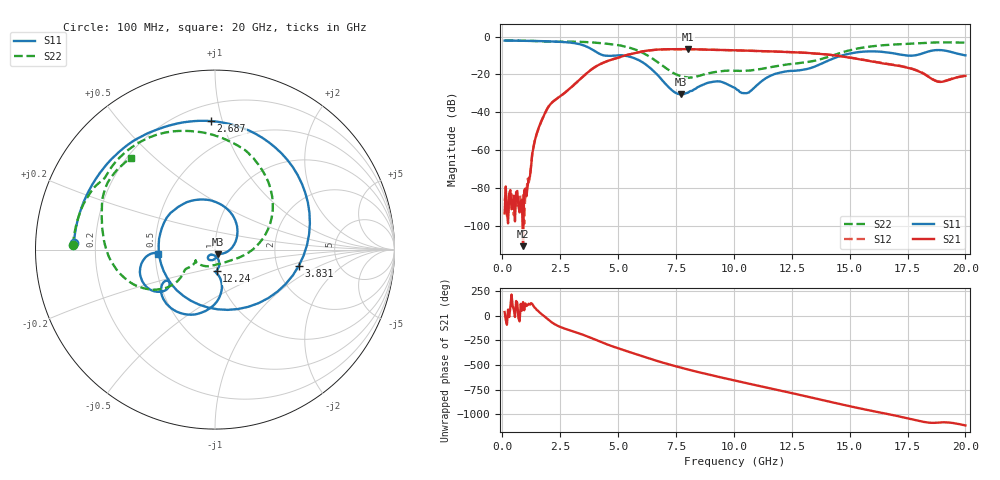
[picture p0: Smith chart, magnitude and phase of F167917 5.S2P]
!  2-Port S-parameters saved by WinCal
! VAR MeasName=S-Parameters (CALIBRATED_DATA) read from VNA (N5242A)
! VAR MeasDate=2016-11-22 8:59:55
! VAR NAME=F167917 5
! VAR FILENAME=F167917 5.S2P
! VAR DATE=2016-11-22 8:59:55
! VAR PHYS_PORTS=1,2
# Hz S DB R 50
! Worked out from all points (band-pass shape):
!   401 points, 100 MHz to 20 GHz, reference 50 ohm
!   highest |S21| = -6.61 dB at 8.01 GHz (marker M1); lowest = -110.9 dB at 896 MHz (marker M2)
!   |S21| within 3 dB of the highest: 5.422 GHz to 14.12 GHz (8.699 GHz wide, 89 % of centre)
!   lowest |S11| = -30.6 dB at 7.712 GHz (marker M3), VSWR 1.06, Z = 51.5 - j2.6 ohm
!   |S11| at or under -10 dB: 4.415 GHz to 4.905 GHz (490 MHz wide, 10.5 % of centre); 5.227 GHz to 14.66 GHz (9.438 GHz wide, 94.9 % of centre); 17.47 GHz to 17.77 GHz (294.6 MHz wide, 1.67 % of centre)
!   |S22| runs from -21.8 to -2.0 dB; largest |S21 - S12| = 0.0047
!   S11 on the Smith chart (normalised r, x): 100 MHz: 0.12, +0.02; 2.687 GHz: 0.31, +0.92; 3.831 GHz: 2.65, -0.61; 12.24 GHz: 0.99, -0.24; 20 GHz: 0.52, -0.03
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1e8  -2.09 177.3  -93.56 36.7  -86.91 -58.3  -2.03 178.3
8.96e8  -2.20 156.1  -110.92 137.7  -84.01 87.9  -2.15 165.6
1.095e9  -2.24 150.5  -79.16 107.8  -75.31 117.9  -2.19 162.4
1.3935e9  -2.29 141.8  -55.70 82.4  -55.48 83.0  -2.30 157.5
1.74175e9  -2.38 130.7  -43.34 6.3  -43.13 5.9  -2.46 151.8
2.687e9  -2.90 91.7  -29.86 -130.4  -29.87 -131.0  -2.63 137.9
3.43325e9  -4.33 37.3  -21.71 170.9  -21.73 170.7  -2.77 122.2
3.83125e9  -6.45 -10.9  -17.56 134.8  -17.56 134.9  -3.01 112.4
4.22925e9  -9.29 -78.1  -14.56 96.0  -14.53 96.1  -3.41 101.9
4.7765e9  -10.11 -171.8  -11.98 47.5  -11.94 47.1  -4.15 85.6
5.52275e9  -10.71 106.9  -9.30 -10.9  -9.31 -11.3  -5.97 56.7
6.7665e9  -21.11 2.2  -6.81 -104.4  -6.84 -104.5  -14.01 -2.3
7.71175e9  -30.61 -58.8  -6.61 -166.8  -6.62 -166.7  -20.93 -52.9
8.01025e9  -29.74 -69.6  -6.61 175.1  -6.61 175.1  -21.64 -74.5
1.005e10  -27.14 -134.0  -7.22 62.0  -7.23 62.0  -18.11 -149.4
1.059725e10  -29.73 -97.9  -7.42 33.5  -7.43 33.4  -18.04 -149.8
1.2239e10  -18.44 -85.6  -8.10 -51.1  -8.09 -51.0  -14.82 -146.1
1.338325e10  -16.36 -81.0  -8.80 -111.6  -8.77 -111.1  -13.02 -142.9
1.4627e10  -10.13 -91.6  -10.42 -178.0  -10.32 -177.8  -8.52 -144.0
1.67165e10  -8.49 -143.1  -14.62 79.7  -14.58 79.5  -4.32 179.3
1.885575e10  -7.10 -158.7  -23.93 -3.6  -23.75 -3.8  -3.03 147.8
2e10  -9.89 -175.8  -20.78 -32.6  -20.67 -33.0  -3.19 132.3
